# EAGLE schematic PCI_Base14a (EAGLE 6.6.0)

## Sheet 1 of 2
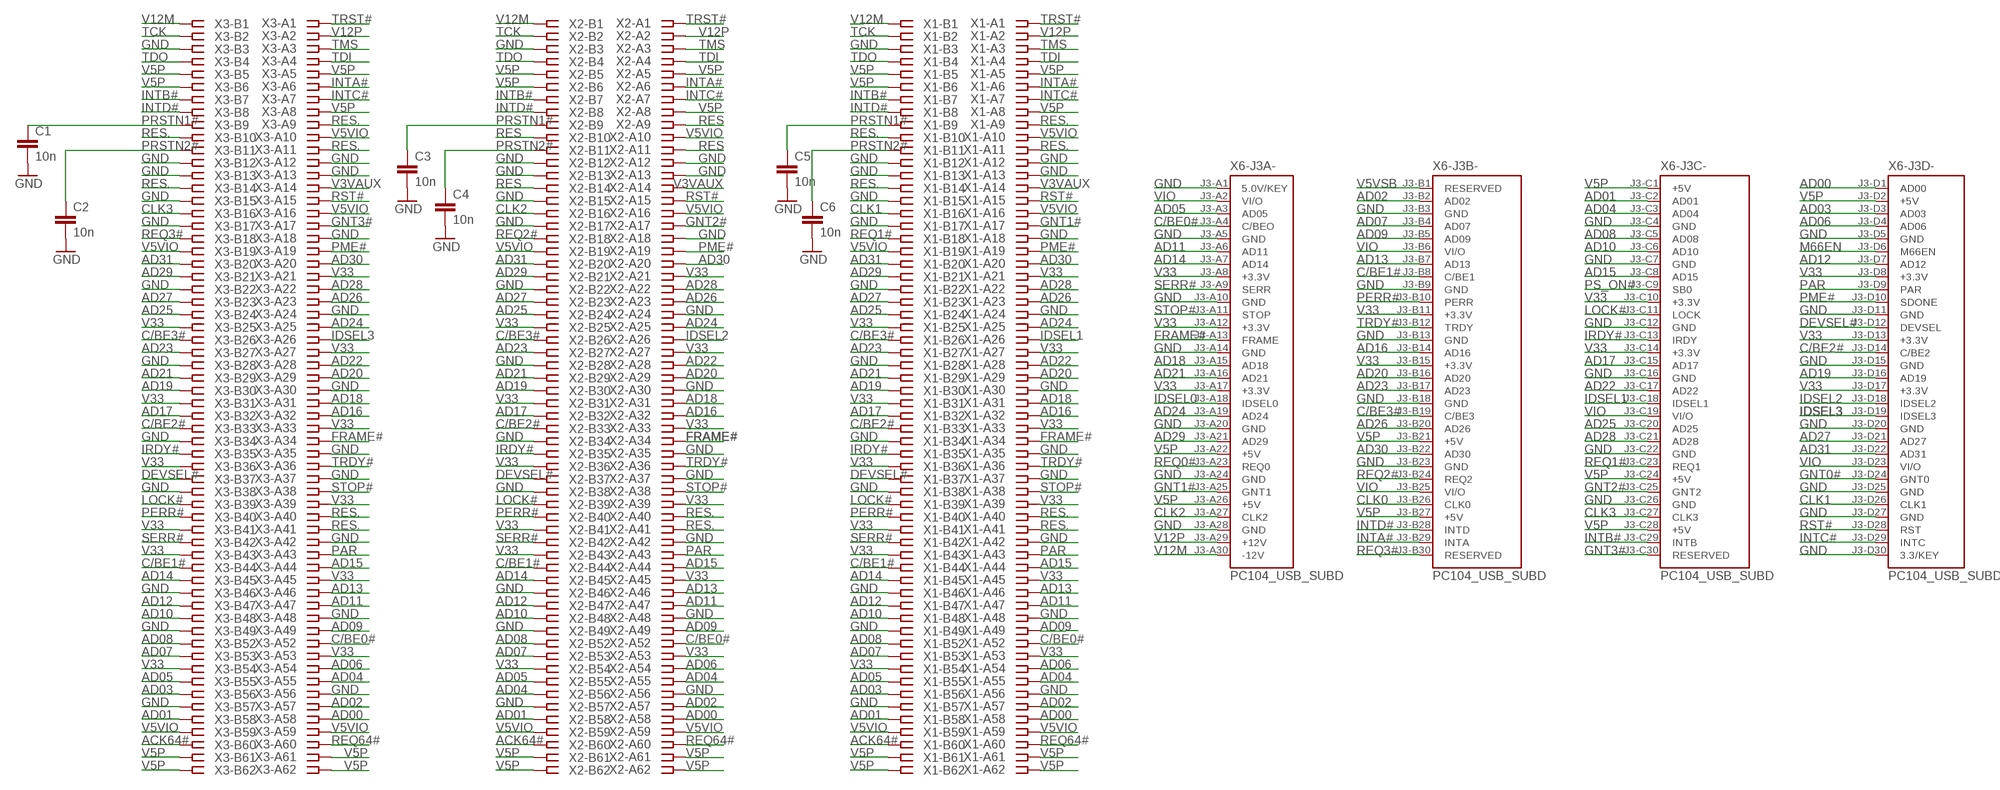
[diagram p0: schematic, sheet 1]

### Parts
C1  10n  C-EUC0805  [C0805]
C2  10n  C-EUC0805  [C0805]
C3  10n  C-EUC0805  [C0805]
C4  10n  C-EUC0805  [C0805]
C5  10n  C-EUC0805  [C0805]
C6  10n  C-EUC0805  [C0805]
X1  PCI-SLOT  [CON-PCI]
X2  PCI-SLOT  [CON-PCI]
X3  PCI-SLOT  [CON-PCI]
X6  PC104_USB_SUBD  [PC104-PLUS]

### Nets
ACK64#: X1.B60 X2.B60 X3.B60 ; also sheet 2
AD00: X1.A58 X2.A58 X3.A58 X6.J3-D1(-J3D-:AD00)
AD01: X1.B58 X2.B58 X3.B58 X6.J3-C2(-J3C-:AD01)
AD02: X1.A57 X2.A57 X3.A57 X6.J3-B2(-J3B-:AD02)
AD03: X1.B56 X3.B56 X6.J3-D3(-J3D-:AD03)
AD04: X1.A55 X2.A55 X2.B56 X3.A55 X6.J3-C3(-J3C-:AD04)
AD05: X1.B55 X2.B55 X3.B55 X6.J3-A3(-J3A-:AD05)
AD06: X1.A54 X2.A54 X3.A54 X6.J3-D4(-J3D-:AD06)
AD07: X1.B53 X2.B53 X3.B53 X6.J3-B4(-J3B-:AD07)
AD08: X1.B52 X2.B52 X3.B52 X6.J3-C5(-J3C-:AD08)
AD09: X1.A49 X2.A49 X3.A49 X6.J3-B5(-J3B-:AD09)
AD10: X1.B48 X2.B48 X3.B48 X6.J3-C6(-J3C-:AD10)
AD11: X1.A47 X2.A47 X3.A47 X6.J3-A6(-J3A-:AD11)
AD12: X1.B47 X2.B47 X3.B47 X6.J3-D7(-J3D-:AD12)
AD13: X1.A46 X2.A46 X3.A46 X6.J3-B7(-J3B-:AD13)
AD14: X1.B45 X2.B45 X3.B45 X6.J3-A7(-J3A-:AD14)
AD15: X1.A44 X2.A44 X3.A44 X6.J3-C8(-J3C-:AD15)
AD16: X1.A32 X2.A32 X3.A32 X6.J3-B14(-J3B-:AD16)
AD17: X1.B32 X2.B32 X3.B32 X6.J3-C15(-J3C-:AD17)
AD18: X1.A31 X2.A31 X3.A31 X6.J3-A15(-J3A-:AD18)
AD19: X1.B30 X2.B30 X3.B30 X6.J3-D16(-J3D-:AD19)
AD20: X1.A29 X2.A29 X3.A29 X6.J3-B16(-J3B-:AD20)
AD21: X1.B29 X2.B29 X3.B29 X6.J3-A16(-J3A-:AD21)
AD22: X1.A28 X2.A28 X3.A28 X6.J3-C17(-J3C-:AD22)
AD23: X1.B27 X2.B27 X3.B27 X6.J3-B17(-J3B-:AD23)
AD24: X1.A25 X2.A25 X3.A25 X6.J3-A19(-J3A-:AD24)
AD25: X1.B24 X2.B24 X3.B24 X6.J3-C20(-J3C-:AD25)
AD26: X1.A23 X2.A23 X3.A23 X6.J3-B20(-J3B-:AD26)
AD27: X1.B23 X2.B23 X3.B23 X6.J3-D21(-J3D-:AD27)
AD28: X1.A22 X2.A22 X3.A22 X6.J3-C21(-J3C-:AD28)
AD29: X1.B21 X2.B21 X3.B21 X6.J3-A21(-J3A-:AD29)
AD30: X1.A20 X2.A20 X3.A20 X6.J3-B22(-J3B-:AD30)
AD31: X1.B20 X2.B20 X3.B20 X6.J3-D22(-J3D-:AD31)
C/BE0#: X1.A52 X2.A52 X3.A52 X6.J3-A4(-J3A-:C/BEO)
C/BE1#: X1.B44 X2.B44 X3.B44 X6.J3-B8(-J3B-:C/BE1)
C/BE2#: X1.B33 X2.B33 X3.B33 X6.J3-D14(-J3D-:C/BE2)
C/BE3#: X1.B26 X2.B26 X3.B26 X6.J3-B19(-J3B-:C/BE3)
CLK0: X6.J3-B26(-J3B-:CLK0)
CLK1: X1.B16 X6.J3-D26(-J3D-:CLK1)
CLK2: X2.B16 X6.J3-A27(-J3A-:CLK2)
CLK3: X3.B16 X6.J3-C27(-J3C-:CLK3)
DEVSEL#: X1.B37 X2.B37 X3.B37 X6.J3-D12(-J3D-:DEVSEL)
FRAME#: X1.A34 X2.A34 X3.A34 X6.J3-A13(-J3A-:FRAME)
GND [supply]: C1.2 C2.2 C3.2 C4.2 C5.2 C6.2 X1.A12 X1.A13 X1.A18 X1.A24 X1.A30 X1.A35 X1.A37 X1.A42 X1.A48 X1.A56 X1.B3 X1.B12 X1.B13 X1.B15 X1.B17 X1.B22 X1.B28 X1.B34 X1.B38 X1.B46 X1.B49 X1.B57 X2.A12 X2.A13 X2.A18 X2.A24 X2.A30 X2.A35 X2.A37 X2.A42 X2.A48 X2.A56 X2.B3 X2.B12 X2.B13 X2.B15 X2.B17 X2.B22 X2.B28 X2.B34 X2.B38 X2.B46 X2.B49 X2.B57 X3.A12 X3.A13 X3.A18 X3.A24 X3.A30 X3.A35 X3.A37 X3.A42 X3.A48 X3.A56 X3.B3 X3.B12 X3.B13 X3.B15 X3.B17 X3.B22 X3.B28 X3.B34 X3.B38 X3.B46 X3.B49 X3.B57 X6.J3-A1(-J3A-:5.0V/KEY) X6.J3-A5(-J3A-:GND) X6.J3-A10(-J3A-:GND) X6.J3-A14(-J3A-:GND) X6.J3-A20(-J3A-:GND) X6.J3-A24(-J3A-:GND) X6.J3-A28(-J3A-:GND) X6.J3-B3(-J3B-:GND) X6.J3-B9(-J3B-:GND) X6.J3-B13(-J3B-:GND) X6.J3-B18(-J3B-:GND) X6.J3-B23(-J3B-:GND) X6.J3-C4(-J3C-:GND) X6.J3-C7(-J3C-:GND) X6.J3-C12(-J3C-:GND) X6.J3-C16(-J3C-:GND) X6.J3-C22(-J3C-:GND) X6.J3-C26(-J3C-:GND) X6.J3-D5(-J3D-:GND) X6.J3-D11(-J3D-:GND) X6.J3-D15(-J3D-:GND) X6.J3-D20(-J3D-:GND) X6.J3-D25(-J3D-:GND) X6.J3-D27(-J3D-:GND) X6.J3-D30(-J3D-:3.3/KEY) ; also sheet 2
GNT0# [supply]: X6.J3-D24(-J3D-:GNT0)
GNT1#: X1.A17 X6.J3-A25(-J3A-:GNT1)
GNT2#: X2.A17 X6.J3-C25(-J3C-:GNT2)
GNT3#: X3.A17 X6.J3-C30(-J3C-:RESERVED)
IDSEL0: X6.J3-A18(-J3A-:IDSEL0)
IDSEL1: X1.A26 X6.J3-C18(-J3C-:IDSEL1)
IDSEL2: X2.A26 X6.J3-D18(-J3D-:IDSEL2)
IDSEL3: X3.A26 X6.J3-D19(-J3D-:IDSEL3)
INTA#: X1.A6 X2.A6 X3.A6 X6.J3-B29(-J3B-:INTA)
INTB#: X1.B7 X2.B7 X3.B7 X6.J3-C29(-J3C-:INTB)
INTC#: X1.A7 X2.A7 X3.A7 X6.J3-D29(-J3D-:INTC)
INTD#: X1.B8 X2.B8 X3.B8 X6.J3-B28(-J3B-:INTD)
IRDY#: X1.B35 X2.B35 X3.B35 X6.J3-C13(-J3C-:IRDY)
LOCK#: X1.B39 X2.B39 X3.B39 X6.J3-C11(-J3C-:LOCK)
M66EN: X6.J3-D6(-J3D-:M66EN)
PAR: X1.A43 X2.A43 X3.A43 X6.J3-D9(-J3D-:PAR)
PERR#: X1.B40 X2.B40 X3.B40 X6.J3-B10(-J3B-:PERR)
PME#: X1.A19 X2.A19 X3.A19 X6.J3-D10(-J3D-:SDONE)
PRSTN1#: C1.1 C3.1 C5.1 X1.B9 X2.B9 X3.B9
PRSTN2#: C2.1 C4.1 C6.1 X1.B11 X2.B11 X3.B11
PS_ON#: X6.J3-C9(-J3C-:SB0) ; also sheet 2
REQ0#: X6.J3-A23(-J3A-:REQ0)
REQ1#: X1.B18 X6.J3-C23(-J3C-:REQ1)
REQ2#: X2.B18 X6.J3-B24(-J3B-:REQ2)
REQ3#: X3.B18 X6.J3-B30(-J3B-:RESERVED)
REQ64#: X1.A60 X2.A60 X3.A60 ; also sheet 2
RES: X2.A9 X2.A11 X2.B10 X2.B14
RES.: X1.A9 X1.A11 X1.A40 X1.A41 X1.B10 X1.B14 X2.A40 X2.A41 X3.A9 X3.A11 X3.A40 X3.A41 X3.B10 X3.B14
RST#: X1.A15 X2.A15 X3.A15 X6.J3-D28(-J3D-:RST)
SERR#: X1.B42 X2.B42 X3.B42 X6.J3-A9(-J3A-:SERR)
STOP#: X1.A38 X2.A38 X3.A38 X6.J3-A11(-J3A-:STOP)
TCK: X1.B2 X2.B2 X3.B2
TDI: X1.A4 X2.A4 X3.A4
TDO: X1.B4 X2.B4 X3.B4
TMS: X1.A3 X2.A3 X3.A3
TRDY#: X1.A36 X2.A36 X3.A36 X6.J3-B12(-J3B-:TRDY)
TRST#: X1.A1 X2.A1 X3.A1
V3VAUX: X1.A14 X2.A14 X3.A14
V5P [supply]: X1.A5 X1.A8 X1.A61 X1.A62 X1.B5 X1.B6 X1.B61 X1.B62 X2.A5 X2.A8 X2.A61 X2.A62 X2.B5 X2.B6 X2.B61 X2.B62 X3.A5 X3.A8 X3.A61 X3.A62 X3.B5 X3.B6 X3.B61 X3.B62 X6.J3-A22(-J3A-:+5V) X6.J3-A26(-J3A-:+5V) X6.J3-B21(-J3B-:+5V) X6.J3-B27(-J3B-:+5V) X6.J3-C1(-J3C-:+5V) X6.J3-C24(-J3C-:+5V) X6.J3-C28(-J3C-:+5V) X6.J3-D2(-J3D-:+5V) ; also sheet 2
V5VIO [supply]: X1.A10 X1.A16 X1.A59 X1.B19 X1.B59 X2.A10 X2.A16 X2.A59 X2.B19 X2.B59 X3.A10 X3.A16 X3.A59 X3.B19 X3.B59 ; also sheet 2
V5VSB: X6.J3-B1(-J3B-:RESERVED)
V12M [supply]: X1.B1 X2.B1 X3.B1 X6.J3-A30(-J3A-:-12V) ; also sheet 2
V12P [supply]: X1.A2 X2.A2 X3.A2 X6.J3-A29(-J3A-:+12V) ; also sheet 2
V33 [supply]: X1.A21 X1.A27 X1.A33 X1.A39 X1.A45 X1.A53 X1.B25 X1.B31 X1.B36 X1.B41 X1.B43 X1.B54 X2.A21 X2.A27 X2.A33 X2.A39 X2.A45 X2.A53 X2.B25 X2.B31 X2.B36 X2.B41 X2.B43 X2.B54 X3.A21 X3.A27 X3.A33 X3.A39 X3.A45 X3.A53 X3.B25 X3.B31 X3.B36 X3.B41 X3.B43 X3.B54 X6.J3-A8(-J3A-:+3.3V) X6.J3-A12(-J3A-:+3.3V) X6.J3-A17(-J3A-:+3.3V) X6.J3-B11(-J3B-:+3.3V) X6.J3-B15(-J3B-:+3.3V) X6.J3-C10(-J3C-:+3.3V) X6.J3-C14(-J3C-:+3.3V) X6.J3-D8(-J3D-:+3.3V) X6.J3-D13(-J3D-:+3.3V) X6.J3-D17(-J3D-:+3.3V) ; also sheet 2
VIO [supply]: X6.J3-A2(-J3A-:VI/O) X6.J3-B6(-J3B-:VI/O) X6.J3-B25(-J3B-:VI/O) X6.J3-C19(-J3C-:VI/O) X6.J3-D23(-J3D-:VI/O) ; also sheet 2

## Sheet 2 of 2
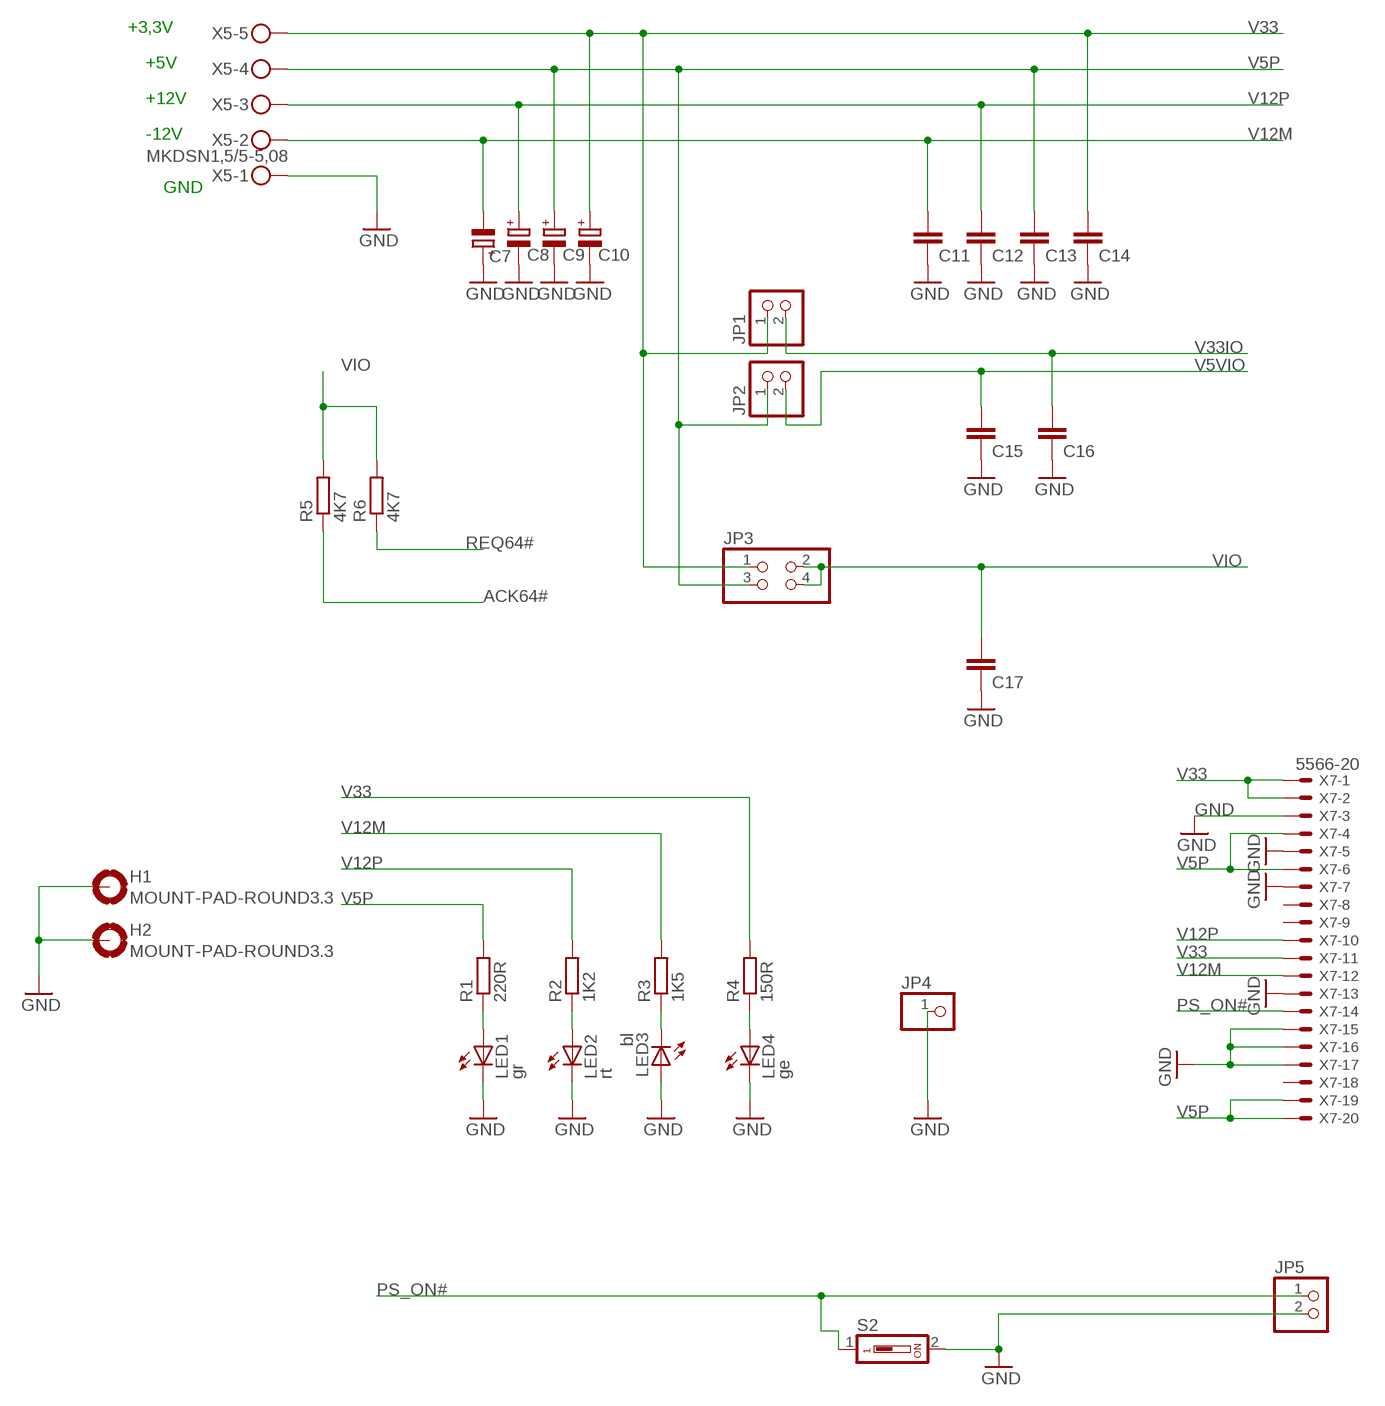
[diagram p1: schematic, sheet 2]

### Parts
C7  47u  CPOL-EUE2.5-5  [E2,5-5]
C8  47u  CPOL-EUE2.5-5  [E2,5-5]
C9  47u  CPOL-EUE2.5-5  [E2,5-5]
C10  47u  CPOL-EUE2.5-5  [E2,5-5]
C11  100n  C-EUC0805  [C0805]
C12  100n  C-EUC0805  [C0805]
C13  100n  C-EUC0805  [C0805]
C14  100n  C-EUC0805  [C0805]
C15  100n  C-EUC0805  [C0805]
C16  100n  C-EUC0805  [C0805]
C17  100n  C-EUC0805  [C0805]
H1  MOUNT-PAD-ROUND3.3  [3,3-PAD]
H2  MOUNT-PAD-ROUND3.3  [3,3-PAD]
JP1  PINHD-1X2  [1X02]
JP2  PINHD-1X2  [1X02]
JP3  PINHD-2X2  [2X02]
JP4  PINHD-1X1  [1X01]
JP5  PINHD-1X2  [1X02]
LED1  gr  LEDSMT1206  [1206]
LED2  rt  LEDSMT1206  [1206]
LED3  bl  LEDSMT1206  [1206]
LED4  ge  LEDSMT1206  [1206]
R1  220R  R-EU_R1206  [R1206]
R2  1K2  R-EU_R1206  [R1206]
R3  1K5  R-EU_R1206  [R1206]
R4  150R  R-EU_R1206  [R1206]
R5  4K7  R-EU_R1206  [R1206]
R6  4K7  R-EU_R1206  [R1206]
S2  DS01  [DS-01]
X5  MKDSN1,5/5-5,08  [MKDSN1,5/5-5,08]
X7  5566-20  [5566-20]

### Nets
ACK64#: R5.1 ; also sheet 1
GND [supply]: C7.+ C8.- C9.- C10.- C11.2 C12.2 C13.2 C14.2 C15.2 C16.2 C17.2 H1.B3,3(MOUNT) H2.B3,3(MOUNT) JP4.1 JP5.2 LED1.C LED2.C LED3.A LED4.C S2.2 X5.1 X7.3 X7.5 X7.7 X7.13 X7.15 X7.16 X7.17 ; also sheet 1
N$1 [supply]: LED4.A R4.1
N$5 [supply]: LED1.A R1.1
N$6 [supply]: LED2.A R2.1
N$7 [supply]: LED3.C R3.1
PS_ON#: JP5.1 S2.1 X7.14 ; also sheet 1
REQ64#: R6.1 ; also sheet 1
V5P [supply]: C9.+ C13.1 JP2.1 JP3.3 R1.2 X5.4 X7.4 X7.6 X7.19 X7.20 ; also sheet 1
V5VIO [supply]: C15.1 JP2.2 ; also sheet 1
V12M [supply]: C7.- C11.1 R3.2 X5.2 X7.12 ; also sheet 1
V12P [supply]: C8.+ C12.1 R2.2 X5.3 X7.10 ; also sheet 1
V33 [supply]: C10.+ C14.1 JP1.1 JP3.1 R4.2 X5.5 X7.1 X7.2 X7.11 ; also sheet 1
V33IO [supply]: C16.1 JP1.2
VIO [supply]: C17.1 JP3.2 JP3.4 R5.2 R6.2 ; also sheet 1
Unconnected: X7.8 X7.9 X7.18

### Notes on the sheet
- +3,3V
- +5V
- +12V
- -12V
- GND

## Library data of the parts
C1-C6 C11-C17 = rcl:C-EU: CAPACITOR, European symbol
C7-C10 = rcl:CPOL-EU: POLARIZED CAPACITOR, European symbol
H1 H2 = holes:MOUNT-PAD-ROUND: MOUNTING PAD, round
JP1 JP2 JP5 = pinhead:PINHD-1X2: PIN HEADER
JP3 = pinhead:PINHD-2X2: PIN HEADER
JP4 = pinhead:PINHD-1X1: PIN HEADER
LED1-LED4 = led:LED: LED
R1-R6 = rcl:R-EU_: RESISTOR, European symbol
S2 = switch-dil:DS01: DIL/CODE SWITCH; OC_FARNELL: unknown; OC_NEWARK: unknown
X1-X3 = con-pc:PCI-SLOT: PCI SLOT
X5 = con-phoenix-508:MKDSN1,5/5-5,08: MKDSN 1,5/ 5-5,08 Printklemme Nennstrom: 13,5 A Nennspannung: 250 V Rastermaß: 5,08 mm Polzahl: 5 Anschlussart: Schraubanschluss Montage: Löten Anschlussrichtung Leiter/Platine: 0 ° Artikelnummer: 1729157 Source: http://eshop.phoenixcontact.com .. 1729157.pdf; MPN: SMKDSN1,5/5-5,08; OC_FARNELL: 1792906; OC_NEWARK: 70R0301
X6 = con-pc104-usb-connector:PC104_USB_SUBD: PC/104-Plus 16 bit
X7 = con-molex:5566-20: Mini FIT connector 20 pol ATX PC-Motherboard Power connector Source: http://www.molex.com; OC_FARNELL: unknown; OC_NEWARK: unknown

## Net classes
0 signal: width 0.305 mm
1 supply: width 0.305 mm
